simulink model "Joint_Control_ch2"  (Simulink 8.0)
settings: Solver=FixedStepDiscrete  SolverMode=SingleTasking  StartTime=0  StopTime=1.2  FixedStep=dt  RelTol=1e-3  SampleTimeConstraint=Specified
InitFcn:
  | % Sampling Times %
  | dt0=0.001; dt1=0.01; samples=10;
undefined symbols (not defined in the file or in its folder): DiscIntNeverNeededParam, Volts
libraries: simulink_extras x6, speedgoatlib_IO311 x3, speedgoatlib_IO101 x2, xpclib x2, simulink x1

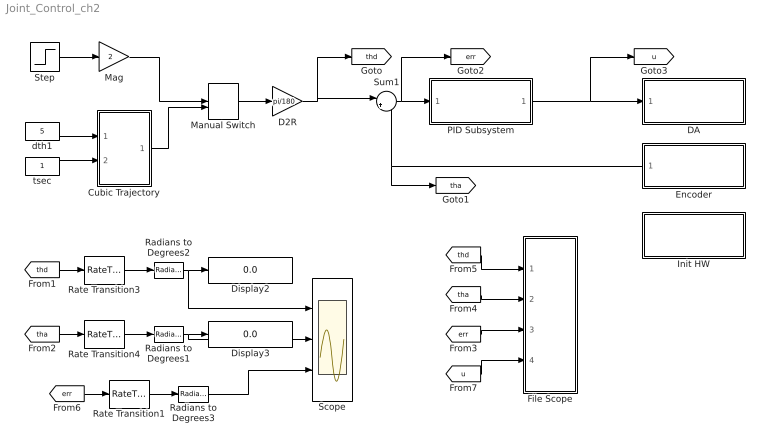
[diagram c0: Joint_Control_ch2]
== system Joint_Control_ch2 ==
  Cubic Trajectory : MATLAB Function  TreatAsAtomicUnit=on
  D2R : Gain  Gain=pi/180  SampleTime=dt0
  DA : Subsystem  TreatAsAtomicUnit=on
  Display2 : Display
  Display3 : Display
  Encoder : Subsystem  TreatAsAtomicUnit=on
  File Scope : Subsystem
  Init HW : Subsystem  TreatAsAtomicUnit=on
  Mag : Gain  Gain=2
  Manual Switch : ManualSwitch
  PID Subsystem : Subsystem  TreatAsAtomicUnit=on
  Radians to Degrees1 : simulink_extras/Transformations/Radians to Degrees
  Radians to Degrees2 : simulink_extras/Transformations/Radians to Degrees
  Radians to Degrees3 : simulink_extras/Transformations/Radians to Degrees
  Rate Transition1 : RateTransition  OutPortSampleTime=dt1
  Rate Transition3 : RateTransition  OutPortSampleTime=dt1
  Rate Transition4 : RateTransition  OutPortSampleTime=dt1
  Scope : Scope  NumInputPorts=3
  Step : Step  Time=0.5  SampleTime=dt0
  Sum1 : Sum  Inputs=|+-
  dth1 : Constant  Value=5
  tsec : Constant
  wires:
  Sum1/1 -> [err], PID Subsystem/1(In1)
  PID Subsystem/1(Out1) -> DA/1(In1), [u]
  [thd] -> Rate Transition3/1
  [tha] -> Rate Transition4/1
  Rate Transition3/1 -> Radians to Degrees2/1
  Rate Transition4/1 -> Radians to Degrees1/1
  Radians to Degrees2/1 -> Display2/1, Scope/1
  Radians to Degrees1/1 -> Display3/1, Scope/2
  [thd] -> File Scope/1(thd)
  [err] -> File Scope/3(err)
  [u] -> File Scope/4(u)
  dth1/1 -> Cubic Trajectory/1(dth)
  tsec/1 -> Cubic Trajectory/2(tsec)
  Step/1 -> Mag/1
  Mag/1 -> Manual Switch/1
  Cubic Trajectory/1(thd) -> Manual Switch/2
  Manual Switch/1 -> D2R/1
  D2R/1 -> [thd], Sum1/1
  Encoder/1(Out1) -> Sum1/2, [tha]
  [tha] -> File Scope/2(tha)
  [err] -> Rate Transition1/1
  Rate Transition1/1 -> Radians to Degrees3/1
  Radians to Degrees3/1 -> Scope/3

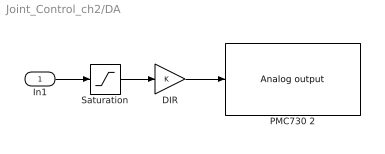
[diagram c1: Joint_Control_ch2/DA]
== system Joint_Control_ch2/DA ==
  In1 : Inport
  DIR : Gain
  PMC730 2 : speedgoatlib_IO101/Analog output  id=1  channel=1  reset=1  initValue=0  ts=dt0  pciSlot=-1
  Saturation : Saturate  UpperLimit=10  LowerLimit=-10
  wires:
  In1/1 -> Saturation/1
  Saturation/1 -> DIR/1
  DIR/1 -> PMC730 2/1

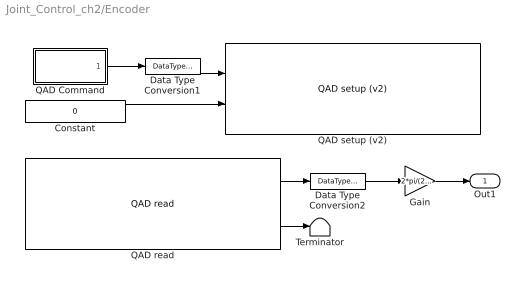
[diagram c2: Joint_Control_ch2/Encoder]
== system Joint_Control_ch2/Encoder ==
  Constant : Constant  Value=0  OutDataTypeStr=Inherit: Inherit via back propagation
  Data Type Conversion1 : DataTypeConversion  OutDataTypeStr=uint8
  Data Type Conversion2 : DataTypeConversion  OutDataTypeStr=double
  Gain : Gain  Gain=2*pi/(23*2000)
  QAD Command : MATLAB Function  TreatAsAtomicUnit=on
  QAD read : speedgoatlib_IO311/QAD/QAD read  id=1  chan=[2]  pciSlot=-1  ts=0.001
  QAD setup (v2) : speedgoatlib_IO311/QAD/QAD setup (v2)  id=1  chan=[2]  debounce=0  quadrature=4x  index=Ignore index input  special=Disabled (cycling counter)  steps=2000  ts=dt0  pciSlot=-1
  Terminator : Terminator
  Out1 : Outport
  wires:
  Gain/1 -> Out1/1
  Constant/1 -> QAD setup (v2)/2
  QAD read/2 -> Terminator/1
  QAD read/1 -> Data Type Conversion2/1
  Data Type Conversion2/1 -> Gain/1
  QAD Command/1(y) -> Data Type Conversion1/1
  Data Type Conversion1/1 -> QAD setup (v2)/1

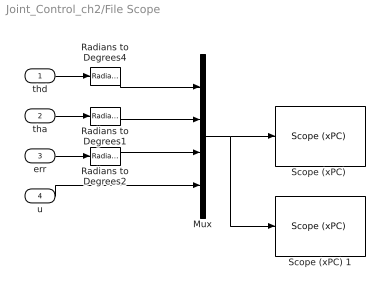
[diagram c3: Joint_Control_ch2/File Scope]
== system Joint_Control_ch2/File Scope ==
  thd : Inport
  tha : Inport  Port=2
  err : Inport  Port=3
  u : Inport  Port=4
  Mux : Mux
  Radians to Degrees1 : simulink_extras/Transformations/Radians to Degrees
  Radians to Degrees2 : simulink_extras/Transformations/Radians to Degrees
  Radians to Degrees4 : simulink_extras/Transformations/Radians to Degrees
  "Scope (xPC) " : xpclib/Misc./Scope (xPC)   scopeno=1  scopetype=File  autostart=on  viewmode=Graphical redraw  formatstr='%15.6f'  grid=on  ylimits=[0,0]  nosamples=100  noprepostsamples=0  interleave=1  triggermode=FreeRun  triggersignal=1  triggerlevel=0.0  triggerslope=Either  triggerscope=1  triggersample=0  filename=step1.dat  mode=Lazy  writesize=512  autorestart=on  dynamicfilemode=off  maxwritefilesize=512*1024^2
  Scope (xPC) 1 : xpclib/Misc./Scope (xPC)   scopeno=2  scopetype=Host  autostart=on  viewmode=Graphical redraw  formatstr='%15.6f'  grid=on  ylimits=[0,0]  nosamples=100  noprepostsamples=0  interleave=1  triggermode=FreeRun  triggersignal=1  triggerlevel=0.0  triggerslope=Either  triggerscope=1  triggersample=0  filename=data1.dat  mode=Lazy  writesize=512  autorestart=off  dynamicfilemode=off  maxwritefilesize=512*1024^2
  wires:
  thd/1 -> Radians to Degrees4/1
  tha/1 -> Radians to Degrees1/1
  err/1 -> Radians to Degrees2/1
  Mux/1 -> "Scope (xPC) "/1, Scope (xPC) 1/1
  Radians to Degrees4/1 -> Mux/1
  Radians to Degrees1/1 -> Mux/2
  Radians to Degrees2/1 -> Mux/3
  u/1 -> Mux/4

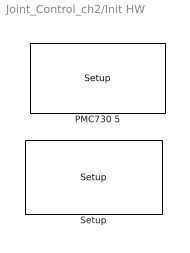
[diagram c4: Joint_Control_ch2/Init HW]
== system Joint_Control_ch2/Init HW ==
  PMC730 5 : speedgoatlib_IO101/Setup  group=Analog output setup  id=1  pciSlot=-1  adStartChannel=1  adNumChannel=1  adCoupling=Single-ended  adRange=-10 .. 10 Volts  adAcqMode=Standard  daChannel=[2]  daReset=[1]  daInitValue=[0]  lowerChannel=1  lowerDirection=Input  lowerDIDebounce=0  lowerDOReset=[1]  lowerDOInitValues=[0]  upperChannel=1  upperDirection=Output  upperDIDebounce=0  upperDOReset=0  upperDOInitValues=0
  Setup : speedgoatlib_IO311/Setup/Setup  group=Module setup  id=1  fpga1=speedgoat_IO311_default  pciSlot=-1  lowerDirection=[1 1 1 1 1 0 0 0 0 0 0 0 1 0 0 0]  lowerReset=[1]  lowerValue=[0]  upperDirection=[1 1 1 1 1 1 1 1 1 0 0 0 0 0 0 0]  upperReset=[1]  upperValue=[0]

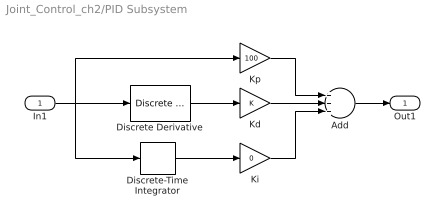
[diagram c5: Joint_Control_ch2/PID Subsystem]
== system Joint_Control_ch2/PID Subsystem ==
  In1 : Inport
  Add : Sum  Inputs=+++
  Discrete Derivative : simulink/Discrete/Discrete Derivative  gainval=1.0  ICPrevScaledInput=0.0  InputProcessing=Inherited  OutMin=[]  OutMax=[]  OutDataType=fixdt(1, 16)  OutScaling=2^-10  DoSatur=off
  Discrete-Time Integrator : DiscreteIntegrator  SampleTime=dt0  ICPrevOutput=DiscIntNeverNeededParam  ICPrevScaledInput=DiscIntNeverNeededParam
  Kd : Gain
  Ki : Gain  Gain=0
  Kp : Gain  Gain=100
  Out1 : Outport
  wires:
  Discrete-Time Integrator/1 -> Ki/1
  Kp/1 -> Add/1
  Kd/1 -> Add/2
  Ki/1 -> Add/3
  Discrete Derivative/1 -> Kd/1
  Add/1 -> Out1/1
  In1/1 -> Kp/1, Discrete Derivative/1, Discrete-Time Integrator/1

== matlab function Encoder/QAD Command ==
function y = fcn()

persistent index

if isempty(index), index=0; end

if index==0
    y=1;      %  Reset %
else
    y = 0;
end

index=index+1;

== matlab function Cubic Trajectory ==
function thd =fcn(dth, tsec)
persistent index thd_p;

if isempty(index), index=0; end
if isempty(thd_p), thd_p=0; end

dt=0.001;

tout=index*dt;
if index<(tsec/dt)
    [c] = coeff_3rd(0, 0, dth, 0, tsec);
    thd=c(1,1)+c(1,2)*tout+c(1,3)*tout^2+c(1,4)*tout^3;    
    thd_p=thd;
else
    thd=thd_p;
end
index=index+1;

function [c] = coeff_3rd(sp, sv, ep, ev, tsec)
MAX_CH=1;
c=zeros(MAX_CH,4);
for ch=1:MAX_CH
    c(ch,1)=sp(ch,1);
    c(ch,2)=sv(ch,1);
    c(ch,3)=(3.0*(ep(ch,1)-sp(ch,1))-(2.0*sv(ch,1)+ev(ch,1))*tsec)/(tsec*tsec);
    c(ch,4)=(-2.0*(ep(ch,1)-sp(ch,1))+(sv(ch,1)+ev(ch,1))*tsec)/(tsec*tsec*tsec);
end
